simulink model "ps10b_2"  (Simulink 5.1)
settings: Solver=ode45  StartTime=0.0  StopTime=10.0  RelTol=1e-3
undefined symbols (not defined in the file or in its folder): Ak, Bk, Ck, Dk

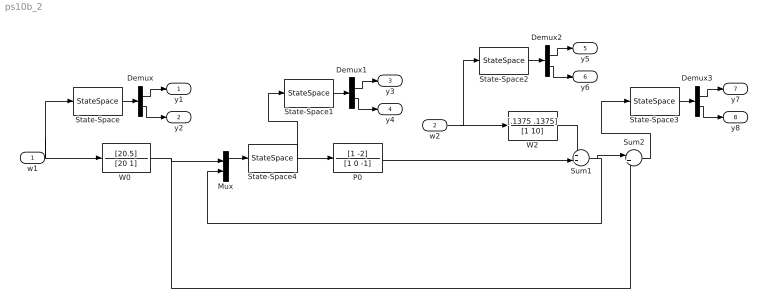
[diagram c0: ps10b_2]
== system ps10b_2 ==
  w1 : Inport
  w2 : Inport  Port=2
  Demux{,1..3} (4 alike) : Demux  Outputs=2
  Mux : Mux  Inputs=2
  P0 : TransferFcn  Numerator=[1 -2]  Denominator=[1 0 -1]
  State-Space{,1..3} (4 alike) : StateSpace  A=-1  C=[1;-1]  D=[0;1]
  State-Space4 : StateSpace  A=Ak  B=Bk  C=Ck  D=Dk
  Sum1 : Sum  Inputs=++|
  Sum2 : Sum  Inputs=|+-
  "W0 " : TransferFcn  Numerator=[20.5]  Denominator=[20 1]
  W2 : TransferFcn  Numerator=[.1375 .1375]  Denominator=[1 10]
  y1 : Outport
  y2 : Outport  Port=2
  y3 : Outport  Port=3
  y4 : Outport  Port=4
  y5 : Outport  Port=5
  y6 : Outport  Port=6
  y7 : Outport  Port=7
  y8 : Outport  Port=8
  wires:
  State-Space/1 -> Demux/1
  w1/1 -> State-Space/1, "W0 "/1
  Demux/1 -> y1/1
  Demux/2 -> y2/1
  "W0 "/1 -> Sum2/2, Mux/1
  State-Space1/1 -> Demux1/1
  Demux1/1 -> y3/1
  Demux1/2 -> y4/1
  State-Space2/1 -> Demux2/1
  Demux2/1 -> y5/1
  Demux2/2 -> y6/1
  w2/1 -> State-Space2/1, W2/1
  W2/1 -> Sum1/1
  P0/1 -> Sum1/2
  Sum1/1 -> Sum2/1, Mux/2
  State-Space3/1 -> Demux3/1
  Demux3/1 -> y7/1
  Demux3/2 -> y8/1
  Sum2/1 -> State-Space3/1
  Mux/1 -> State-Space4/1
  State-Space4/1 -> State-Space1/1, P0/1
